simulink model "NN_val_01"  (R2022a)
settings: Solver=VariableStepAuto  StartTime=0.0  StopTime=300  RelTol=1e-3
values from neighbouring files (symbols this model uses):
  C = 6.3000e-04    (= 0.00063)    [maglev_init.m]
  g = 9.80    (= 9.8)    [maglev_init.m]
  K = 1.0e+03 * [-2.4567   -0.1235    0.0237]    [maglev_init.m]
  L1 = 0.6000    (= 0.6)    [maglev_init.m]
  m = 0.0300    (= 0.03)    [maglev_init.m]
  mpert = 0    [maglev_init.m]
  R = 45    [maglev_init.m]
  Ts = 0.005    [maglev_init.m]    (also in train_net.m)
  x1_0 = 0.1    [maglev_init.m]
  x1_d = 0.05    [maglev_init.m]
  x2_0 = 0    [maglev_init.m]
  x2_d = 0    [maglev_init.m]
  x3_0 = 0.2    [maglev_init.m]
undefined symbols (not defined in the file or in its folder): magnitude
libraries: neural x10

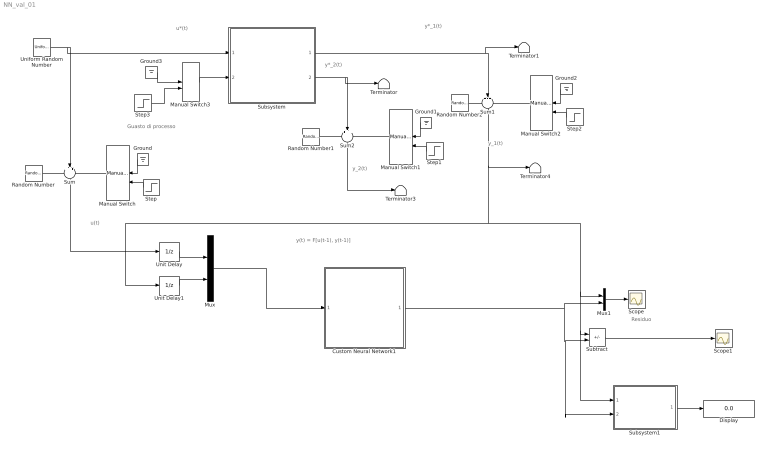
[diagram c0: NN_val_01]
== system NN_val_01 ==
  note: Residuo
  note: y(t) = F[u(t-1), y(t-1)]
  note: y_2(t)
  note: y*_1(t)
  note: u(t)
  note: y*_2(t)
  note: y_1(t)
  note: u*(t)
  note: Guasto di processo
  Custom Neural Network1 : Subsystem
      mask help: Custom Neural Network
  Display : Display
  Ground{,1..3} (4 alike) : Ground
  Manual Switch{,1..3} (4 alike) : ManualSwitch
  Mux : Mux  Inputs=2
  Mux1 : Mux  Inputs=2
  Random Number : RandomNumber  Variance=1e-9  Seed=1  SampleTime=Ts
  Random Number1 : RandomNumber  Variance=1e-6  Seed=3  SampleTime=Ts
  Random Number2 : RandomNumber  Variance=1e-9  Seed=2  SampleTime=Ts
  Scope : Scope
  Scope1 : Scope
  Step : Step  Time=150  SampleTime=0
  Step1 : Step  Time=150  SampleTime=0
  Step2 : Step  Time=150  SampleTime=0
  Step3 : Step  Time=15  After=2*R  SampleTime=0
  Subsystem : Subsystem
  Subsystem1 : Subsystem
  Subtract : Sum  Inputs=+-
  Sum : Sum  Inputs=+++
  Sum1 : Sum  Inputs=+++
  Sum2 : Sum  Inputs=+++
  Terminator{,1,3..4} (4 alike) : Terminator
  Uniform Random Number : UniformRandomNumber  Minimum=x1_d*0.9  Maximum=x1_d*1.1  Seed=1  SampleTime=0.5
  Unit Delay : UnitDelay  SampleTime=Ts  HasFrameUpgradeWarning=on
  Unit Delay1 : UnitDelay  SampleTime=Ts  HasFrameUpgradeWarning=on
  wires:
  Subsystem/1(Out1) -> Terminator1/1, Sum1/2
  Subsystem/2(Out2) -> Terminator/1, Sum2/2
  Random Number/1 -> Sum/1
  Manual Switch/1 -> Sum/3
  Manual Switch2/1 -> Sum1/3
  Manual Switch1/1 -> Sum2/3
  Random Number1/1 -> Sum2/1
  Ground/1 -> Manual Switch/1
  Step/1 -> Manual Switch/2
  Ground1/1 -> Manual Switch1/1
  Step1/1 -> Manual Switch1/2
  Sum2/1 -> Terminator3/1
  Random Number2/1 -> Sum1/1
  Ground2/1 -> Manual Switch2/1
  Step2/1 -> Manual Switch2/2
  Manual Switch3/1 -> Subsystem/2(fs)
  Ground3/1 -> Manual Switch3/1
  Uniform Random Number/1 -> Subsystem/1(u), Sum/2
  Step3/1 -> Manual Switch3/2
  Sum/1 -> Unit Delay/1
  Unit Delay/1 -> Mux/1
  Unit Delay1/1 -> Mux/2
  Mux/1 -> Custom Neural Network1/1(Input)
  Custom Neural Network1/1(Output) -> Mux1/2, Subsystem1/2(y_prev), Subtract/2
  Subtract/1 -> Scope1/1
  Mux1/1 -> Scope/1
  Sum1/1 -> Terminator4/1, Subsystem1/1(y_mis), Subtract/1, Mux1/1, Unit Delay1/1
  Subsystem1/1(VAF%) -> Display/1

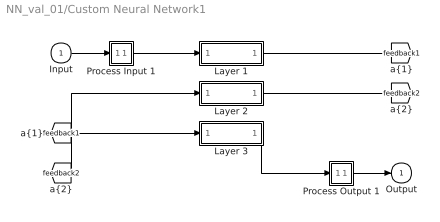
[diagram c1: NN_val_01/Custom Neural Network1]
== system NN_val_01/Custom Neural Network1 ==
  Input : Inport  PortDimensions=2  SampleTime=0.005
  Layer 1 : Subsystem
  Layer 2 : Subsystem
  Layer 3 : Subsystem
  Process Input 1 : Subsystem
  Process Output 1 : Subsystem
  Output : Outport  InitialOutput=0
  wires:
  Layer 3/1("a{3}") -> Process Output 1/1(a)
  [feedback2] -> Layer 3/1("a{2} ")
  Layer 2/1("a{2}") -> [feedback2]
  [feedback1] -> Layer 2/1("a{1} ")
  Layer 1/1("a{1}") -> [feedback1]
  Process Input 1/1(p) -> Layer 1/1("p{1}")
  Process Output 1/1(y) -> Output/1
  Input/1 -> Process Input 1/1(x)

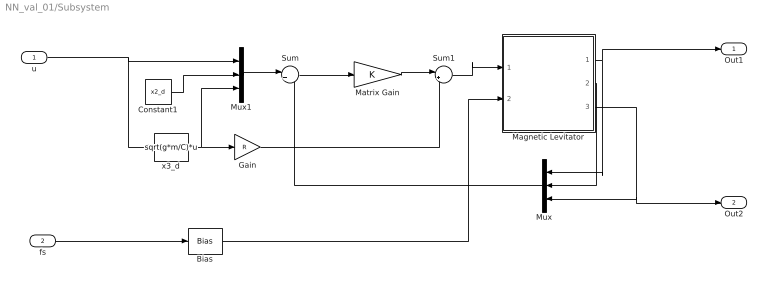
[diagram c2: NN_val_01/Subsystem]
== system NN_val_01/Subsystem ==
  u : Inport
  fs : Inport  Port=2
  Bias : Bias  Bias=R
  Constant1 : Constant  Value=x2_d
  Gain : Gain  Gain=R
  Magnetic Levitator : Subsystem  mask{m=m+mpert, R=R, L1=L1, C=C, g=g}
      mask prompts: m "ball's mass (m)"; R "Electromagnet's resistance (R)"; L1 "Electromagnet's inductance (L1)"; C "Magnetic force constant (C)"; g "Gravitational acceleration (g)"
  Matrix Gain : Gain  Gain=K  Multiplication=Matrix(K*u)  SaturateOnIntegerOverflow=on
  Mux : Mux  Inputs=3
  Mux1 : Mux  Inputs=3
  Sum : Sum  Inputs=|+-  InputSameDT=on  SaturateOnIntegerOverflow=on
  Sum1 : Sum  Inputs=|++  InputSameDT=on  SaturateOnIntegerOverflow=on
  x3_d : Fcn  Expr=sqrt(g*m/C)*u
  Out1 : Outport
  Out2 : Outport  Port=2
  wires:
  u/1 -> x3_d/1, Mux1/1
  Magnetic Levitator/2(x2) -> Mux/2
  x3_d/1 -> Mux1/3, Gain/1
  Mux1/1 -> Sum/1
  Gain/1 -> Sum1/2
  Mux/1 -> Sum/2
  Constant1/1 -> Mux1/2
  Sum/1 -> Matrix Gain/1
  Sum1/1 -> Magnetic Levitator/1(u)
  Magnetic Levitator/1(x1) -> Out1/1, Mux/1
  Magnetic Levitator/3(x3) -> Out2/1, Mux/3
  Matrix Gain/1 -> Sum1/1
  Bias/1 -> Magnetic Levitator/2(fs)
  fs/1 -> Bias/1

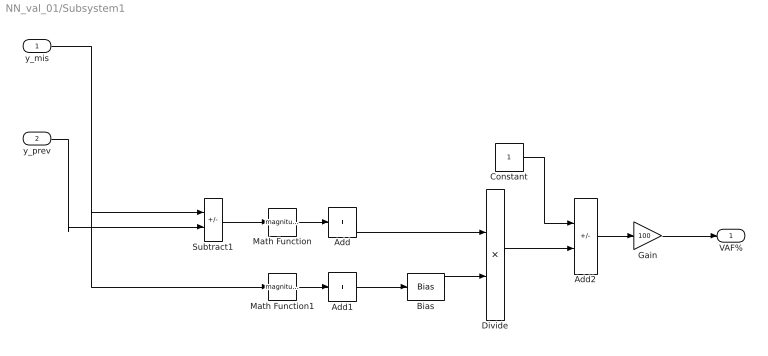
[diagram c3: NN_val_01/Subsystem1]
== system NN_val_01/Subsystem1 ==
  y_mis : Inport
  y_prev : Inport  Port=2
  Add : Sum  Inputs=+
  Add1 : Sum  Inputs=+
  Add2 : Sum  Inputs=+-
  Bias : Bias  Bias=1e-7
  Constant : Constant
  Divide : Product  Inputs=*/
  Gain : Gain  Gain=100
  Math Function : Math  Operator=magnitude^2
  Math Function1 : Math  Operator=magnitude^2
  Subtract1 : Sum  Inputs=+-
  VAF% : Outport
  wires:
  Add2/1 -> Gain/1
  Math Function/1 -> Add/1
  Bias/1 -> Divide/2
  y_mis/1 -> Math Function1/1, Subtract1/1
  Add1/1 -> Bias/1
  Math Function1/1 -> Add1/1
  Subtract1/1 -> Math Function/1
  Constant/1 -> Add2/1
  Divide/1 -> Add2/2
  Add/1 -> Divide/1
  y_prev/1 -> Subtract1/2
  Gain/1 -> VAF%/1

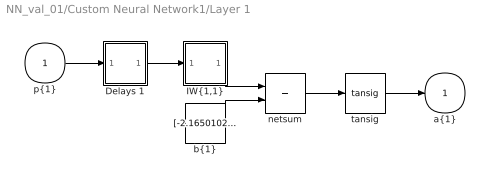
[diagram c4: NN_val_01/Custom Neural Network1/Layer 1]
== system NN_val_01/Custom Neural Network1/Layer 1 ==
  "p{1}" : Inport  PortDimensions=2  SampleTime=0.005
  Delays 1 : Subsystem
  "IW{1,1}" : Subsystem
  "b{1}" : Constant  Value=[-2.165010232984565075042837634100578725337982177734375;-0.99018084463472033629471980020753107964992523193359375]
  netsum : Sum  Inputs=2  InputSameDT=on  SaturateOnIntegerOverflow=on
  tansig : neural/Transfer Functions/tansig
  "a{1}" : Outport  InitialOutput=[0;0]
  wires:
  tansig/1 -> "a{1}"/1
  netsum/1 -> tansig/1
  "b{1}"/1 -> netsum/2
  "IW{1,1}"/1("iz{1,1}") -> netsum/1
  Delays 1/1("pd{1,1}") -> "IW{1,1}"/1("pd{1,1}")
  "p{1}"/1 -> Delays 1/1("p{1}")

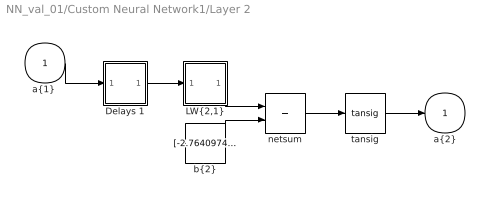
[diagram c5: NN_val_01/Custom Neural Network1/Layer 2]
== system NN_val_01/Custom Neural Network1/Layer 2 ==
  "a{1} " : Inport  PortDimensions=2  SampleTime=0.005
  Delays 1 : Subsystem
  "LW{2,1}" : Subsystem
  "b{2}" : Constant  Value=[-2.76409742947160541604034733609296381473541259765625;0.91391405324340713178798978333361446857452392578125;-0.79693396570784413857069239384145475924015045166015625;2.83340357653886432132139816530980169773101806640625]
  netsum : Sum  Inputs=2  InputSameDT=on  SaturateOnIntegerOverflow=on
  tansig : neural/Transfer Functions/tansig
  "a{2}" : Outport  InitialOutput=[0;0;0;0]
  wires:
  tansig/1 -> "a{2}"/1
  netsum/1 -> tansig/1
  "b{2}"/1 -> netsum/2
  "LW{2,1}"/1("lz{2,1}") -> netsum/1
  Delays 1/1("pd{2,1}") -> "LW{2,1}"/1("ad{2,1}")
  "a{1} "/1 -> Delays 1/1("p{2}")

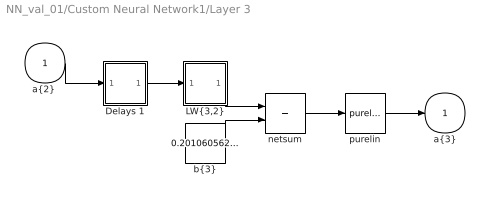
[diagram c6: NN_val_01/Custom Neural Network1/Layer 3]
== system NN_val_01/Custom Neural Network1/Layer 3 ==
  "a{2} " : Inport  PortDimensions=4  SampleTime=0.005
  Delays 1 : Subsystem
  "LW{3,2}" : Subsystem
  "b{3}" : Constant  Value=0.2010605623167778244209102922468446195125579833984375
  netsum : Sum  Inputs=2  InputSameDT=on  SaturateOnIntegerOverflow=on
  purelin : neural/Transfer Functions/purelin
  "a{3}" : Outport  InitialOutput=0
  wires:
  purelin/1 -> "a{3}"/1
  netsum/1 -> purelin/1
  "b{3}"/1 -> netsum/2
  "LW{3,2}"/1("lz{3,2}") -> netsum/1
  Delays 1/1("pd{3,2}") -> "LW{3,2}"/1("ad{3,2}")
  "a{2} "/1 -> Delays 1/1("p{3}")

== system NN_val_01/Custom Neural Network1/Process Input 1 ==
  x : Inport  PortDimensions=2  SampleTime=0.005
  p : Outport  PortDimensions=2  SampleTime=0.005
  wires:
  x/1 -> p/1

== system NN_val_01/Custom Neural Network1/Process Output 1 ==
  a : Inport  PortDimensions=1  SampleTime=0.005
  y : Outport  PortDimensions=1  SampleTime=0.005
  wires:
  a/1 -> y/1

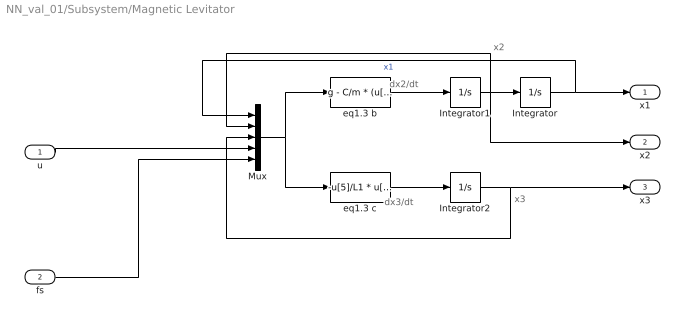
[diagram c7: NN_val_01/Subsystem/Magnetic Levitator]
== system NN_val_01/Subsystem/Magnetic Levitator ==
  note: x2
  note: x3
  note: dx2/dt
  note: dx3/dt
  u : Inport
  fs : Inport  Port=2
  Integrator : Integrator  InitialCondition=x1_0
  Integrator1 : Integrator  InitialCondition=x2_0
  Integrator2 : Integrator  InitialCondition=x3_0
  Mux : Mux  Inputs=5
  eq1.3 b : Fcn  Expr=g - C/m * (u[3] / u[1])^2
  eq1.3 c : Fcn  Expr=-u[5]/L1 * u[3] + (2*C)/L1 * ( u[2] * u[3] / u[1]^2 ) + 1/L1 * u[4]
  x1 : Outport
  x2 : Outport  Port=2
  x3 : Outport  Port=3
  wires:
  eq1.3 b/1 -> Integrator1/1
  Integrator1/1 -> Integrator/1, Mux/2, x2/1
  eq1.3 c/1 -> Integrator2/1
  Mux/1 -> eq1.3 b/1, eq1.3 c/1
  Integrator/1 -> Mux/1, x1/1  "x1"
  Integrator2/1 -> Mux/3, x3/1
  u/1 -> Mux/4
  fs/1 -> Mux/5

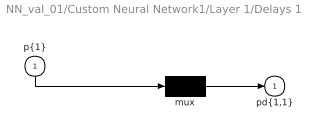
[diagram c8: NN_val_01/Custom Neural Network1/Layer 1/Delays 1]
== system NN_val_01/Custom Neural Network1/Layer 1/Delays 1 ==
  "p{1}" : Inport  PortDimensions=2  SampleTime=0.005
  mux : Mux  Inputs=1
  "pd{1,1}" : Outport
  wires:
  mux/1 -> "pd{1,1}"/1
  "p{1}"/1 -> mux/1

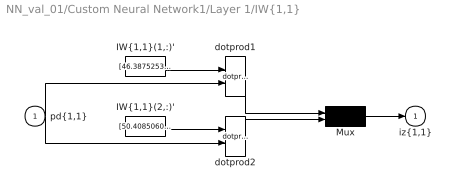
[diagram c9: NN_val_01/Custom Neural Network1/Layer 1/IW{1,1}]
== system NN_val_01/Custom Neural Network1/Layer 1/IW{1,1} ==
  "pd{1,1}" : Inport  PortDimensions=2  SampleTime=0.005
  "IW{1,1}(1,:)'" : Constant  Value=[46.38752532641807846403025905601680278778076171875;-30.02020716206245509738437249325215816497802734375]
  "IW{1,1}(2,:)'" : Constant  Value=[50.408506029134514392353594303131103515625;28.00458439829532153453328646719455718994140625]
  Mux : Mux  Inputs=2
  dotprod1 : neural/Weight Functions/dotprod
  dotprod2 : neural/Weight Functions/dotprod
  "iz{1,1}" : Outport
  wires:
  Mux/1 -> "iz{1,1}"/1
  dotprod2/1 -> Mux/2
  "IW{1,1}(2,:)'"/1 -> dotprod2/1
  dotprod1/1 -> Mux/1
  "pd{1,1}"/1 -> dotprod2/2, dotprod1/2
  "IW{1,1}(1,:)'"/1 -> dotprod1/1

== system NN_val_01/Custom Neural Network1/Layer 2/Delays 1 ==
  "p{2}" : Inport  PortDimensions=2  SampleTime=0.005
  mux : Mux  Inputs=1
  "pd{2,1}" : Outport
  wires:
  mux/1 -> "pd{2,1}"/1
  "p{2}"/1 -> mux/1

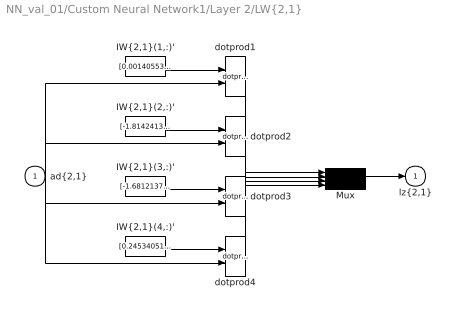
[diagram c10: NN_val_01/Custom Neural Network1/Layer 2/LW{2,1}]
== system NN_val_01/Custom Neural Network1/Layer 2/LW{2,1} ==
  "ad{2,1}" : Inport  PortDimensions=2  SampleTime=0.005
  "IW{2,1}(1,:)'" : Constant  Value=[0.001405533007920074795027431946436990983784198760986328125;2.76441434699151766807290186989121139049530029296875]
  "IW{2,1}(2,:)'" : Constant  Value=[-1.8142413042354241792253333187545649707317352294921875;2.12830136073460085555097975884564220905303955078125]
  "IW{2,1}(3,:)'" : Constant  Value=[-1.6812137832937150694334604850155301392078399658203125;-2.2096304124726291462366134510375559329986572265625]
  "IW{2,1}(4,:)'" : Constant  Value=[0.245340519136751533668672209387295879423618316650390625;2.76382363851122736519982936442829668521881103515625]
  Mux : Mux
  dotprod{1..4} (4 alike) : neural/Weight Functions/dotprod
  "lz{2,1}" : Outport
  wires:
  Mux/1 -> "lz{2,1}"/1
  dotprod4/1 -> Mux/4
  "IW{2,1}(4,:)'"/1 -> dotprod4/1
  dotprod3/1 -> Mux/3
  "IW{2,1}(3,:)'"/1 -> dotprod3/1
  dotprod2/1 -> Mux/2
  "IW{2,1}(2,:)'"/1 -> dotprod2/1
  dotprod1/1 -> Mux/1
  "ad{2,1}"/1 -> dotprod4/2, dotprod3/2, dotprod2/2, dotprod1/2
  "IW{2,1}(1,:)'"/1 -> dotprod1/1

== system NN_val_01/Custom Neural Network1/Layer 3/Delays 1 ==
  "p{3}" : Inport  PortDimensions=4  SampleTime=0.005
  mux : Mux  Inputs=1
  "pd{3,2}" : Outport
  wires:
  mux/1 -> "pd{3,2}"/1
  "p{3}"/1 -> mux/1

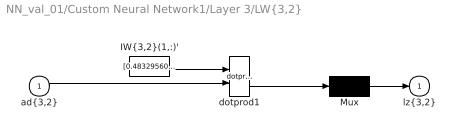
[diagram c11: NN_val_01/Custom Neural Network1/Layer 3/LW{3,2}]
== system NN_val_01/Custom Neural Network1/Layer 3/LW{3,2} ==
  "ad{3,2}" : Inport  PortDimensions=4  SampleTime=0.005
  "IW{3,2}(1,:)'" : Constant  Value=[0.483295609205659226770279701668187044560909271240234375;0.356104986175123150449195463806972838938236236572265625;0.2319393811096205626487432027715840376913547515869140625;-0.2873034152097859728058892869739793241024017333984375]
  Mux : Mux  Inputs=1
  dotprod1 : neural/Weight Functions/dotprod
  "lz{3,2}" : Outport
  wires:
  Mux/1 -> "lz{3,2}"/1
  dotprod1/1 -> Mux/1
  "ad{3,2}"/1 -> dotprod1/2
  "IW{3,2}(1,:)'"/1 -> dotprod1/1
